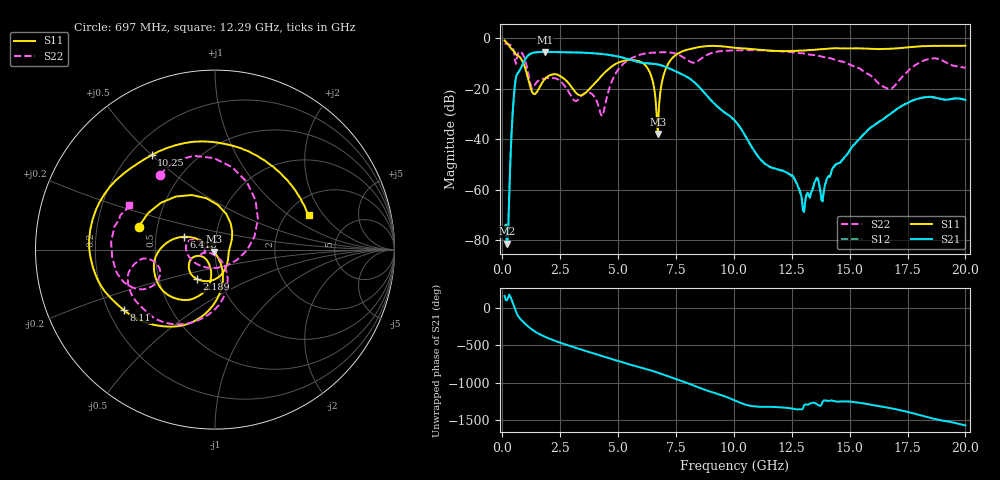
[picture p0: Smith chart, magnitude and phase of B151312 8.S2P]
!  2-Port S-parameters saved by WinCal
! VAR MeasName=S-Parameters (CALIBRATED_DATA) read from VNA (N5244A)
! VAR MeasDate=12/8/2015 5:44:17 PM
! VAR NAME=B151312 8
! VAR FILENAME=B151312 8.S2P
! VAR DATE=12/8/2015 5:44:17 PM
! VAR PHYS_PORTS=1,2
# Hz S DB R 50
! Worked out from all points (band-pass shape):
!   401 points, 100 MHz to 20 GHz, reference 50 ohm
!   highest |S21| = -5.45 dB at 1.841 GHz (marker M1); lowest = -81.4 dB at 199.5 MHz (marker M2)
!   |S21| within 3 dB of the highest: 987.8 MHz to 5.494 GHz (4.507 GHz wide, 139 % of centre)
!   lowest |S11| = -38.0 dB at 6.717 GHz (marker M3), VSWR 1.03, Z = 49.6 - j1.2 ohm
!   |S11| at or under -10 dB: 913.2 MHz to 4.936 GHz (4.023 GHz wide, 138 % of centre); 6.09 GHz to 7.177 GHz (1.086 GHz wide, 16.4 % of centre)
!   |S22| runs from -30.9 to -2.2 dB; largest |S21 - S12| = 0.0014
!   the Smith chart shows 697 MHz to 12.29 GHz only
!   S11 on the Smith chart (normalised r, x): 697 MHz: 0.39, +0.12; 2.189 GHz: 0.78, -0.27; 6.418 GHz: 0.70, +0.10; 8.11 GHz: 0.26, -0.28; 10.25 GHz: 0.28, +0.50; 12.29 GHz: 2.60, +1.45
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1e8  -0.90 -41.8  -76.90 155.9  -75.08 118.0  -2.19 169.3
1.995e8  -1.91 -77.0  -81.41 98.0  -82.44 115.1  -2.28 158.2
4.98e8  -5.09 -156.8  -23.33 28.7  -23.34 28.6  -5.25 108.3
6.97e8  -7.05 163.3  -13.52 -119.2  -13.52 -119.3  -5.69 126.4
1.24425e9  -20.29 22.2  -6.06 76.1  -6.06 76.1  -19.14 -53.3
1.84125e9  -16.16 -83.1  -5.45 -28.3  -5.45 -28.3  -15.94 -177.6
2.1895e9  -14.33 -121.0  -5.51 -72.5  -5.51 -72.6  -15.77 169.4
3.43325e9  -22.59 -129.1  -5.73 158.5  -5.72 158.5  -22.62 -157.6
4.32875e9  -14.50 -98.6  -6.29 72.7  -6.29 72.7  -30.87 -102.4
4.92575e9  -10.04 -117.2  -7.12 16.0  -7.12 16.0  -13.52 -70.8
6.41825e9  -14.63 157.2  -10.06 -116.6  -10.06 -116.6  -5.79 -134.7
6.71675e9  -37.95 -107.8  -10.42 -146.8  -10.44 -146.8  -5.66 -143.6
6.7665e9  -27.00 -69.8  -10.53 -152.1  -10.54 -152.0  -5.62 -144.8
7.1645e9  -10.19 -91.9  -11.81 165.5  -11.77 165.5  -5.60 -155.8
8.10975e9  -4.31 -146.2  -16.14 61.1  -16.12 61.0  -9.31 -167.9
1.005e10  -3.82 131.6  -32.75 -158.3  -32.81 -158.5  -4.83 -175.0
1.0249e10  -3.96 123.8  -35.07 175.5  -35.15 175.3  -4.81 -177.6
1.228875e10  -5.10 20.2  -53.33 104.1  -53.16 102.9  -5.41 152.7
1.298525e10  -4.88 -15.0  -68.37 95.1  -66.70 101.6  -6.02 143.6
1.338325e10  -4.67 -32.2  -60.49 167.3  -59.82 169.5  -6.67 138.0
1.67165e10  -4.21 -111.2  -30.32 103.0  -30.15 102.8  -20.09 160.2
2e10  -2.99 -147.2  -24.48 -130.2  -24.49 -131.3  -11.81 126.2
